VAR_GLOBAL
	ipCreator: I_AcsiCodeCreatorClass := GVL_AcsiVars.Creator.SetCodeRev(codeRev:=3).SetGuiVer(major:=1, minor:=1, build:=94, revision:=4);
	fbIED: FB_IED_IED;
	(* User defined clock (time stamp source) *)
	fbMyClock : FB_MyClock;
	{warning 'Please configure your server IP-address in the initialization code of the server function block below:'}
	(* Server container *)
	fbIEDServer: FB_iec61850ServerClass := (ipIED:=fbIED, ipSystemClock:=fbMyClock, settings:=(bEnable:=TRUE, sLocalHost:='127.0.0.1'));
	
	(* Server connections *)
	fbIEDServerSession1: FB_IEDServerSession := (fbConnection:=(ipServer:=fbIEDServer, settings:=(bEnable:=TRUE)));
	(*	
	fbIEDServerSession2: FB_IEDServerSession := (fbConnection:=(ipServer:=fbIEDServer, settings:=(bEnable:=TRUE)));
	...
	fbIEDServerSessionN: FB_IEDServerSession := (fbConnection:=(ipServer:=fbIEDServer, settings:=(bEnable:=TRUE)));
	*)
END_VAR
